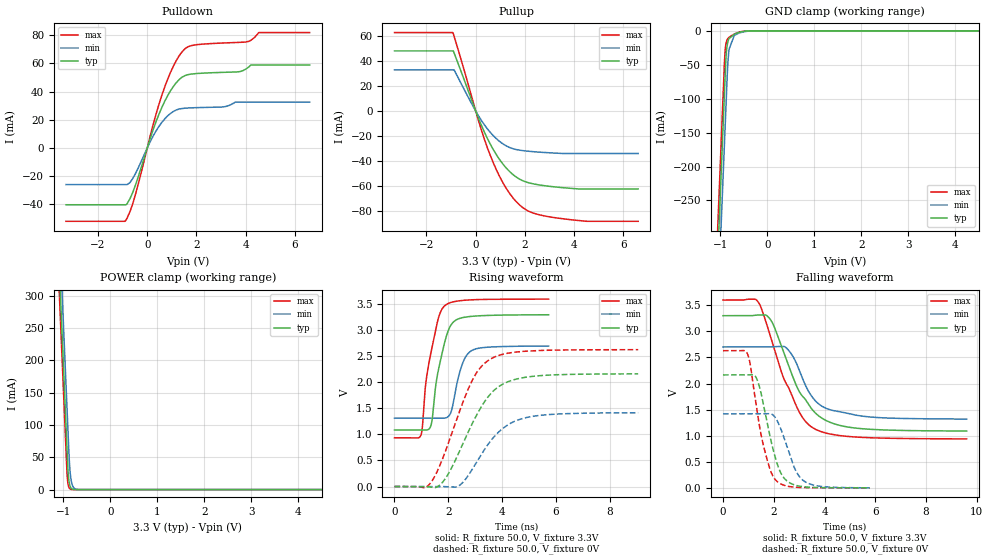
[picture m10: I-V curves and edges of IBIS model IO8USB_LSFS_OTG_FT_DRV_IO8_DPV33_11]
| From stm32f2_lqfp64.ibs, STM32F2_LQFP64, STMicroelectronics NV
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| *** New cell (Generated with 5.14beta1 (Sep 20 2010 13:23:23))
[Model]   IO8USB_LSFS_OTG_FT_DRV_IO8_DPV33_11
Model_type 3-state
Polarity   Non-Inverting
Enable   Active-Low
| CAP_THRESHOLD on pad DPV33 is "CMOS" :
| Rising=10.0% of vddio   Falling=90.0% of vddio
| C_comp min and max val. don't necessarily correlate with the min and max pvt
| but are the smallest and greatest pad capacitance found.
| var   typ   min   max
C_comp   5.85475pF  5.58530pF  6.39105pF
Vmeas = 1.65V   | Reference voltage for timing measurements
Cref  = 400.0pF   | Timing specification test load capacitance value
Rref  = 1.0MOhm   | Timing specification test load resistance value
Vref  = 1.65V   | Timing specification test load voltage
[Model Spec]
| variable   typ   min   max
[Temperature Range] 25.0 125.0 -40.0
| variable   typ   min   max
[Voltage Range] 3.3V 2.7V 3.6V
| variable   typ   min   max
[POWER Clamp Reference] 3.3V 2.7V 3.6V
| variable   typ   min   max
[GND Clamp Reference] 0V 0V 0V
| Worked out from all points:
|   slope of the pulldown table from 0 to 0.495 V, typ, clamps not added: 20 ohm
|   slope of the pullup table from 0 to 0.495 V, typ, clamps not added: 21.7 ohm
|   GND clamp passes 1 mA (typ) near -0.51 V on its own axis
|   POWER clamp passes 1 mA (typ) near -0.81 V on its own axis
|   rising waveform, R_fixture 50.0, V_fixture 3.3V: 20-80 % time 460ps typ, 397ps min, 469ps max; typ from 1.09 V to 3.3 V
|   falling waveform, R_fixture 50.0, V_fixture 3.3V: 20-80 % time 1.27ns typ, 950ps min, 1.22ns max; typ from 3.3 V to 1.09 V
|   rising waveform, R_fixture 50.0, V_fixture 0V: 20-80 % time 1.3ns typ, 1.24ns min, 1.17ns max; typ from 0 V to 2.16 V
|   falling waveform, R_fixture 50.0, V_fixture 0V: 20-80 % time 619ps typ, 643ps min, 592ps max; typ from 2.17 V to 0 V
[POWER Clamp]
-3.3V     4.11A      4.173A     4.072A
-1.09V    352.5mA    415.9mA    314.5mA
-1.05V    284.5mA    347.9mA    246.5mA
-1.01V    216.5mA    279.9mA    178.5mA
-920mV    63.51mA    126.9mA    25.85mA
-900mV    31.51mA    92.9mA     9.552mA
-890mV    21.35mA    75.9mA     5.807mA
-870mV    9.804mA    44.01mA    2.146mA
-840mV    3.05mA     18.36mA    482.1uA
-780mV    295.2uA    3.193mA    24.34uA
-660mV    2.775uA    96uA       63.85nA
6.6V      0A         0A         0A
[GND Clamp]
-3.3V     -4.155A    -4.23A     -4.11A
-1.06V    -347.4mA   -421.9mA   -301.9mA
-940mV    -143.4mA   -217.9mA   -97.86mA
-910mV    -92.43mA   -166.9mA   -46.86mA
-890mV    -58.43mA   -132.9mA   -25.36mA
-880mV    -43.4mA    -115.9mA   -20.1mA
-860mV    -25.79mA   -81.93mA   -14.41mA
-840mV    -17.12mA   -51.2mA    -11.69mA
-820mV    -12.64mA   -32.88mA   -10.09mA
-700mV    -5.102mA   -6.6mA     -4.73mA
-230mV    -826nA     -13.68uA   -47.8nA
6.6V      45.45nA    5.674uA    302.2pA
| variable   typ   min   max
[Pullup Reference] 3.3V 2.7V 3.6V
| variable   typ   min   max
[Pulldown Reference] 0V 0V 0V
[Pullup]
-3.3V     48.28mA    33.1mA     63mA
-930mV    48.28mA    33.1mA     63mA
-880mV    46.73mA    33.1mA     60.07mA
120mV     -6.142mA   -4.065mA   -8.189mA
590mV     -26.5mA    -17.07mA   -35.52mA
1.18V     -44.36mA   -27.27mA   -60.11mA
1.54V     -51.43mA   -30.39mA   -70.35mA
1.89V     -55.75mA   -31.69mA   -77.18mA
2.48V     -58.98mA   -32.83mA   -82.75mA
3.6V      -61.62mA   -34.07mA   -86.61mA
4.51V     -62.54mA   -34.07mA   -88.51mA
6.6V      -62.54mA   -34.07mA   -88.51mA
[Pulldown]
-3.3V     -40.26mA   -25.94mA   -51.99mA
-870mV    -40.25mA   -25.94mA   -51.33mA
-700mV    -35.92mA   -24.51mA   -45.06mA
-470mV    -25.89mA   -17.87mA   -32.39mA
240mV     12.97mA    8.52mA     16.62mA
590mV     28.62mA    18.11mA    37.2mA
1.07V     43.85mA    26mA       58.31mA
1.54V     51.42mA    28.24mA    70.48mA
2.01V     52.82mA    28.63mA    73.27mA
4.01V     56.01mA    32.56mA    75.18mA
4.53V     58.89mA    32.56mA    81.88mA
6.6V      58.89mA    32.56mA    81.88mA
[Ramp]
dV/dt_r 1.29849V/1.29676ns 850.49043mV/1.24038ns 1.57707V/1.17229ns
dV/dt_f 1.3266V/1.2715ns 829.53356mV/949.88323ps 1.59711V/1.22073ns
R_load = 50.0
| Removed startup time: 0s 0s 0s  .
| Removed end time: 5.726ns.
[Rising Waveform]
R_fixture   = 50.0
V_fixture   = 3.3V
V_fixture_min = 2.7V
V_fixture_max = 3.6V
0s        1.087V     1.314V     936.3mV
981ps     1.087V     1.314V     985.7mV
1.166ns   1.084V     1.314V     1.998V
1.364ns   1.189V     1.314V     2.596V
1.569ns   2.066V     1.314V     3.107V
1.857ns   2.754V     1.313V     3.469V
2.181ns   3.156V     1.599V     3.547V
2.494ns   3.24V      2.312V     3.573V
2.821ns   3.267V     2.596V     3.586V
5.728ns   3.3V       2.699V     3.6V
| Removed startup time: 0s 0s 0s  .
| Removed end time: 9.598ns.
[Falling Waveform]
R_fixture   = 50.0
V_fixture   = 3.3V
V_fixture_min = 2.7V
V_fixture_max = 3.6V
0s        3.3V       2.7V       3.6V
1.38ns    3.313V     2.7V       3.567V
1.896ns   3.206V     2.703V     2.863V
2.483ns   2.479V     2.688V     2.006V
2.985ns   1.864V     2.281V     1.473V
3.31ns    1.648V     1.905V     1.243V
3.601ns   1.454V     1.69V      1.134V
4.091ns   1.284V     1.518V     1.046V
5.125ns   1.151V     1.404V     977.9mV
9.6ns     1.089V     1.317V     938.1mV
| Removed startup time: 0s 0s 0s  .
| Removed end time: 9.052ns.
[Rising Waveform]
R_fixture   = 50.0
V_fixture   = 0V
V_fixture_min = 0V
V_fixture_max = 0V
0s        17.05nV    1.21uV     10.93nV
1.12ns    73.07uV    -4.139uV   -25.66mV
1.348ns   -11.15mV   22.88uV    74.11mV
1.809ns   96.2mV     -929.6uV   563mV
2.439ns   706mV      31.81mV    1.475V
2.998ns   1.32V      424.5mV    2.143V
3.586ns   1.789V     885mV      2.455V
4.198ns   2.009V     1.18V      2.559V
5.01ns    2.109V     1.337V     2.604V
9.054ns   2.164V     1.417V     2.628V
| Removed startup time: 0s 0s 0s  .
| Removed end time: 5.78ns.
[Falling Waveform]
R_fixture   = 50.0
V_fixture   = 0V
V_fixture_min = 0V
V_fixture_max = 0V
0s        2.165V     1.419V     2.629V
969ps     2.165V     1.419V     2.563V
1.079ns   2.168V     1.419V     2.351V
1.389ns   2.016V     1.419V     1.334V
1.778ns   1.158V     1.423V     475.5mV
2.1ns     516.9mV    1.318V     137.5mV
2.469ns   154.9mV    870.8mV    40.34mV
2.843ns   52.86mV    353.1mV    12.82mV
3.187ns   20.99mV    132.8mV    5.43mV
5.782ns   274.7uV    580.8uV    222.8uV
